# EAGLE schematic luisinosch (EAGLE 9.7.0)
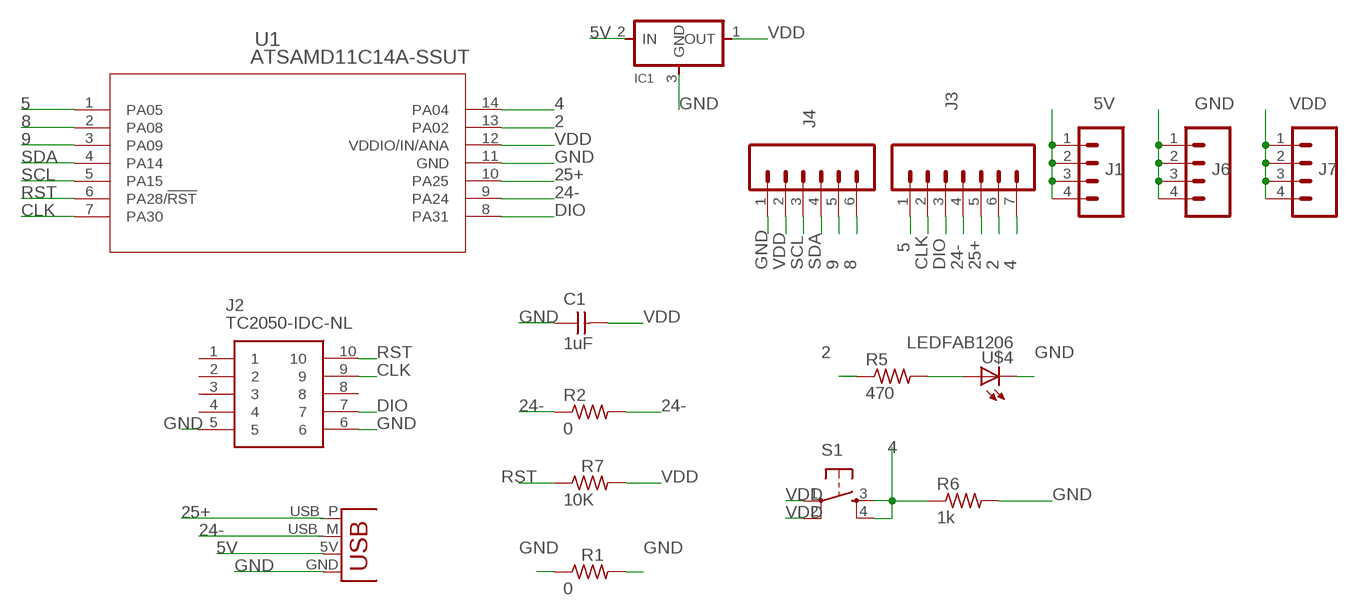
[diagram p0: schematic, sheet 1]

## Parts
C1  1uF  CAP_UNPOLARIZEDFAB  [C1206FAB]
IC1  VR_REGULATOR-SOT23SOT23  [SOT23]
J1  CONN_04LONGPADS  [1X04_LONGPADS]
J2  TC2050-IDC-NL  [TC2050IDCNL]
J3  CONN_07LONGPADS  [1X07_LONGPADS]
J4  CONN_06LONGPADS  [1X06_LONGPADS]
J6  CONN_04LONGPADS  [1X04_LONGPADS]
J7  CONN_04LONGPADS  [1X04_LONGPADS]
R1  0  R1206FAB  [R1206FAB]
R2  0  R1206FAB  [R1206FAB]
R5  470  R1206FAB  [R1206FAB]
R6  1k  RES-US1206FAB  [R1206FAB]
R7  10K  R1206FAB  [R1206FAB]
S1  SW_SWITCH_TACTILE_6MM6MM_SWITCH  [6MM_SWITCH]
U1  ATSAMD11C14A-SSUT  [SOIC14_SL_MCH]
U$4  LEDFAB1206  [LED1206FAB]
X1  CONN_USBPCB  [USB-A-PCB]

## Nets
2: J3.6 R5.1 U1.13(PA02)
4: J3.7 R6.1 S1.3(S) S1.4(S1) U1.14(PA04)
5: J3.1 U1.1(PA05)
5V: IC1.2(IN) J1.1 J1.2 J1.3 J1.4 X1.5V(VBUS)
8: J4.6 U1.2(PA08)
9: J4.5 U1.3(PA09)
24-: J3.4 R2.1 R2.2 U1.9(PA24) X1.USB_M(D-)
25+: J3.5 U1.10(PA25) X1.USB_P(D+)
CLK: J2.9 J3.2 U1.7(PA30)
DIO: J2.7 J3.3 U1.8(PA31)
GND: C1.1 IC1.3(GND) J2.5 J2.6 J4.1 J6.1 J6.2 J6.3 J6.4 R1.1 R1.2 R6.2 U1.11(GND) U$4.2(C) X1.GND
N$5: R5.2 U$4.1(A)
RST: J2.10 R7.1 U1.6(PA28/!RST)
SCL: J4.3 U1.5(PA15)
SDA: J4.4 U1.4(PA14)
VDD: C1.2 IC1.1(OUT) J4.2 J7.1 J7.2 J7.3 J7.4 R7.2 S1.1(P) S1.2(P1) U1.12(VDDIO/IN/ANA)
Unconnected: J2.1 J2.2 J2.3 J2.4 J2.8

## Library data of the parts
C1 = fab:CAP_UNPOLARIZED
IC1 = fab:VR_REGULATOR-SOT23
J1 J6 J7 = SparkFun-Connectors:CONN_04: Multi connection point. Often used as Generic Header-pin footprint for 0.1 inch spaced/style header connections On any of the 0.1 inch spaced packages, you can populate with these: Break Away Headers - Straight (PRT-00116) Break Away Male Headers - Right Angle (PRT-00553) Female Headers (PRT-00115)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; PROD_ID: CONN-09696
J2 = TC2050-IDC-NL:TC2050-IDC-NL: 10-Pin No-Legs Plug-of-Nails Cable with Ribbon connector. CBL PLUG-OF-NAILS 10-PIN Source: Datasheet; DESCRIPTION: 10-Pin No-Legs Plug-of-Nails Cable with Ribbon connector. CBL PLUG-OF-NAILS 10-PIN; HEIGHT: 29.66mm; MANUFACTURER_NAME: Tag-Connect; MANUFACTURER_PART_NUMBER: TC2050-IDC-NL
J3 = SparkFun-Connectors:CONN_07: Multi connection point. Often used as Generic Header-pin footprint for 0.1 inch spaced/style header connections On any of the 0.1 inch spaced packages, you can populate with these: Break Away Headers - Straight (PRT-00116) Break Away Male Headers - Right Angle (PRT-00553) Female Headers (PRT-00115)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
J4 = SparkFun-Connectors:CONN_06: Multi connection point. Often used as Generic Header-pin footprint for 0.1 inch spaced/style header connections On any of the 0.1 inch spaced packages, you can populate with these: Break Away Headers - Straight (PRT-00116) Break Away Male Headers - Right Angle (PRT-00553) Female Headers (PRT-00115)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
R1 R2 R5 R7 = fab:R: Resistor (US Symbol)
R6 = fab:RES-US: Resistor (US Symbol)
S1 = fab:SW_SWITCH_TACTILE_6MM: OMRON SWITCH
U1 = samd11c:ATSAMD11C14A-SSUT; BUILT_BY: EMA_Molly; COPYRIGHT: Copyright (C) 2018 Accelerated Designs. All rights reserved; MANUFACTURER_PART_NUMBER: ATSAMD11C14A-SSUT; SOURCELIBRARY: Microchip_2019-08-23_25; VENDOR: Microchip
U$4 = fab:LED: LED
X1 = fab:CONN_USB: USB Connectors USB-B-PTH is fully proven SKU : PRT-00139 USB-miniB is fully proven SKU : PRT-00587 USB-A-PCB is untested. USB-A-H is throughly reviewed, but untested. Spark Fun Electronics SKU : PRT-00437 USB-B-SMT is throughly reviewed, but untested. Needs silkscreen touching up. USB-A-S has not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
